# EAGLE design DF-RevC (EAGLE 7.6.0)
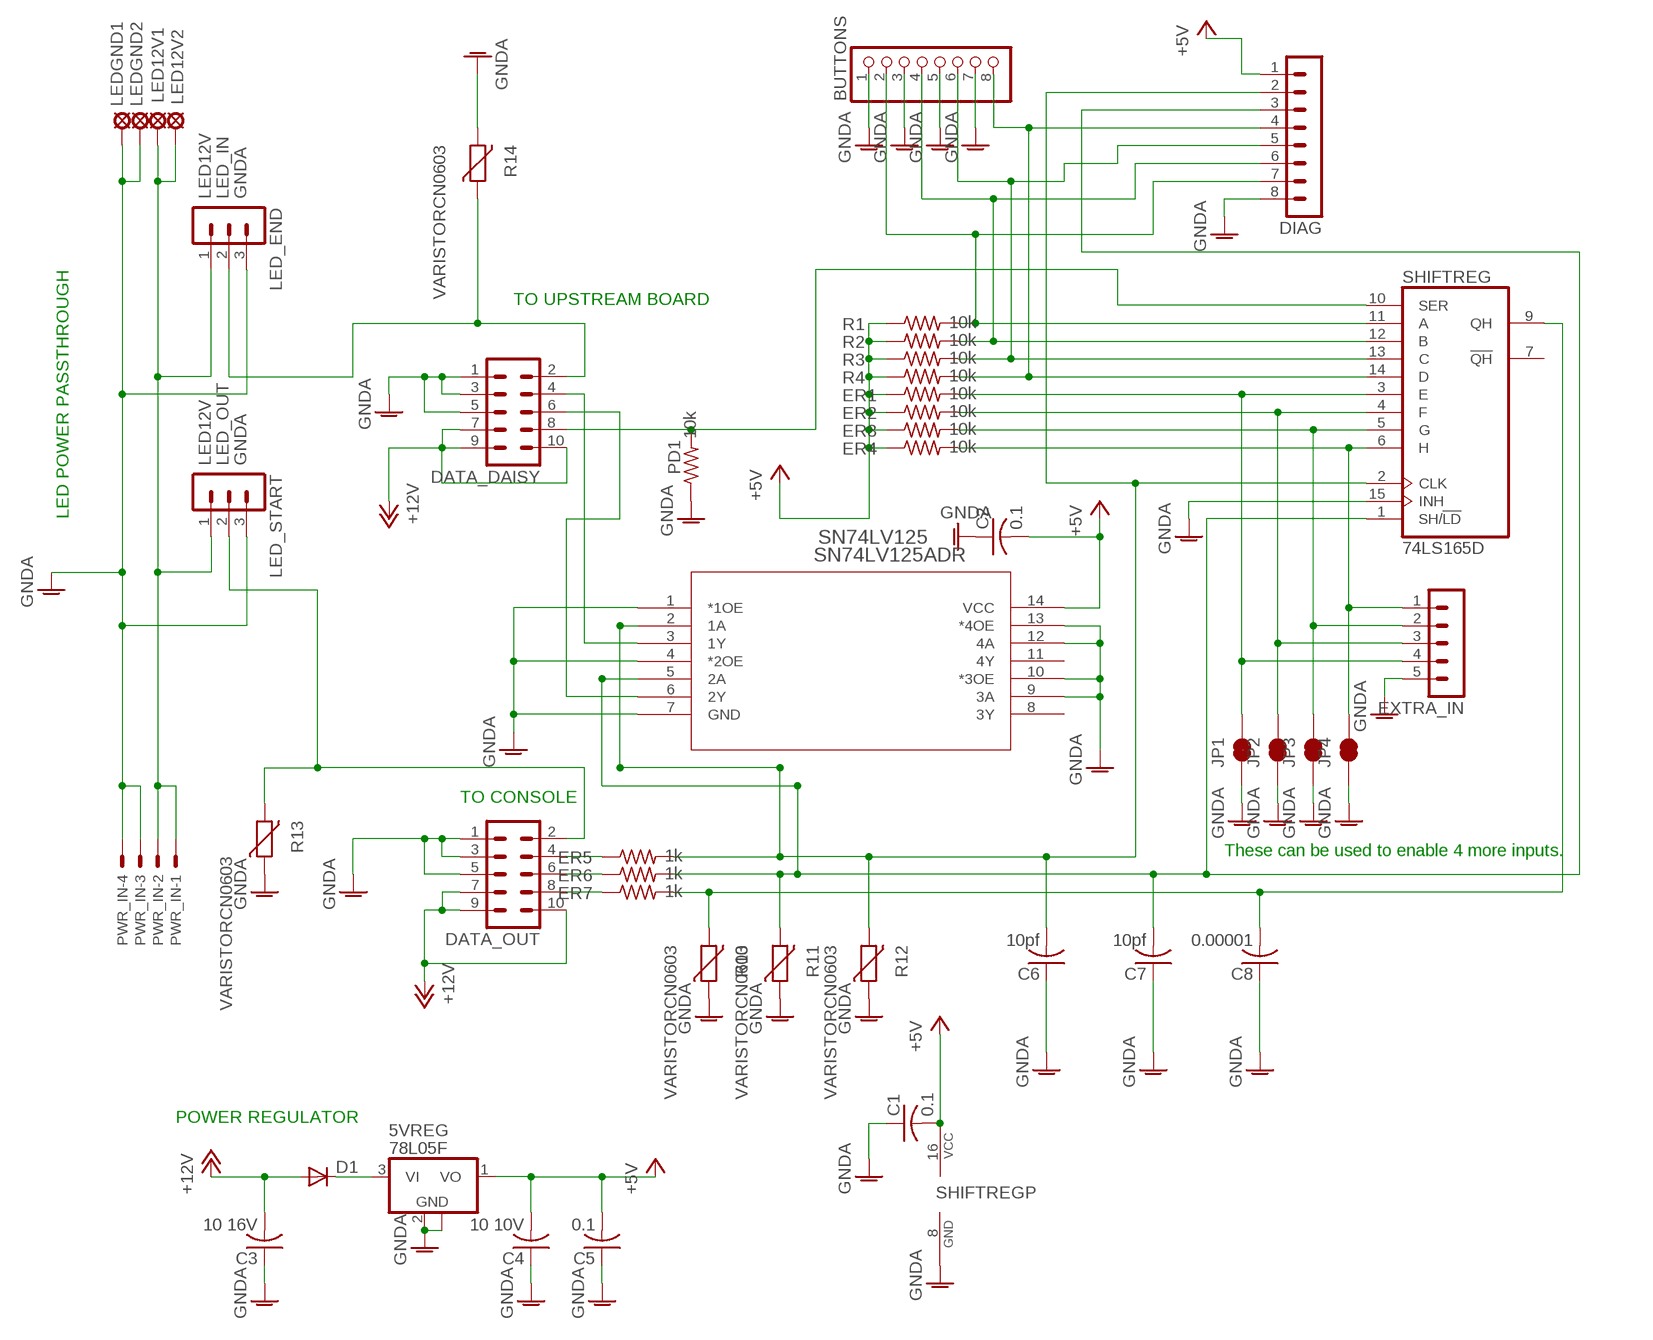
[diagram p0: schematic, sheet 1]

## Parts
5VREG  78L05F  [SOT89]
BUTTONS  SPRING-TERMINAL_8/PTSA-ZZ_2.5MM  [1X8/PTSA-ZZ_2.5MM]
C1  0.1  C-USC0603  [C0603]
C2  0.1  C-USC0603  [C0603]
C3  10 16V  C-USC0603  [C0603]
C4  10 10V  C-USC0603  [C0603]
C5  0.1  C-USC0603  [C0603]
C6  10pf  C-USC0603  [C0603]
C7  10pf  C-USC0603  [C0603]
C8  0.00001  C-USC0603  [C0603]
D1  DIODE-SOD323-R  [SOD323-R]
DATA_DAISY  MA05-2  [MA05-2]
DATA_OUT  MA05-2  [MA05-2]
DIAG  MA08-1  [MA08-1]
ER1  10k  R-US_R0603  [R0603]
ER2  10k  R-US_R0603  [R0603]
ER3  10k  R-US_R0603  [R0603]
ER4  10k  R-US_R0603  [R0603]
ER5  1k  R-US_R0603  [R0603]
ER6  1k  R-US_R0603  [R0603]
ER7  1k  R-US_R0603  [R0603]
EXTRA_IN  MA05-1  [MA05-1]
JP1  JUMPER-PAD-2-NC_BY_TRACE  [PAD-JUMPER-2-NC_BY_TRACE_YES_SILK]
JP2  JUMPER-PAD-2-NC_BY_TRACE  [PAD-JUMPER-2-NC_BY_TRACE_YES_SILK]
JP3  JUMPER-PAD-2-NC_BY_TRACE  [PAD-JUMPER-2-NC_BY_TRACE_YES_SILK]
JP4  JUMPER-PAD-2-NC_BY_TRACE  [PAD-JUMPER-2-NC_BY_TRACE_YES_SILK]
LED12V1  SE14  [SE14]
LED12V2  SE14  [SE14]
LED_END  MA03-1  [MA03-1]
LED_START  MA03-1  [MA03-1]
LEDGND1  SE14  [SE14]
LEDGND2  SE14  [SE14]
PD1  10k  R-US_R0603  [R0603]
PWR_IN  KK-156-4  [KK-156-4]
R1  10k  R-US_R0603  [R0603]
R2  10k  R-US_R0603  [R0603]
R3  10k  R-US_R0603  [R0603]
R4  10k  R-US_R0603  [R0603]
R10  VARISTORCN0603  [CT/CN0603]
R11  VARISTORCN0603  [CT/CN0603]
R12  VARISTORCN0603  [CT/CN0603]
R13  VARISTORCN0603  [CT/CN0603]
R14  VARISTORCN0603  [CT/CN0603]
SHIFTREG  74LS165D  [SO16]
SN74LV125  SN74LV125ADR  [D14]

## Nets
+5V: 5VREG.1(VO) C1.2 C2.2 C4.2 C5.2 DIAG.1 ER1.1 ER2.1 ER3.1 ER4.1 R1.1 R2.1 R3.1 R4.1 SHIFTREG.16(VCC) SN74LV125.14(VCC)
+12V: C3.2 D1.A DATA_DAISY.7 DATA_DAISY.9 DATA_DAISY.10 DATA_OUT.7 DATA_OUT.9 DATA_OUT.10
CLK: C6.2 DIAG.2 ER5.2 R12.2 SHIFTREG.2(CLK) SN74LV125.2(1A)
GNDA: 5VREG.2(GND) 5VREG.2@1(GND) BUTTONS.1 BUTTONS.3 BUTTONS.5 BUTTONS.7 C1.1 C2.1 C3.1 C4.1 C5.1 C6.1 C7.1 C8.1 DATA_DAISY.1 DATA_DAISY.3 DATA_DAISY.5 DATA_OUT.1 DATA_OUT.3 DATA_OUT.5 DIAG.8 EXTRA_IN.5 JP1.1 JP2.1 JP3.1 JP4.1 LED_END.3 LED_START.3 LEDGND1.MP LEDGND2.MP PD1.1 PWR_IN.3 PWR_IN.4 R10.1 R11.1 R12.1 R13.1 R14.2 SHIFTREG.8(GND) SHIFTREG.15(INH) SN74LV125.1(*1OE) SN74LV125.4(*2OE) SN74LV125.7(GND) SN74LV125.9(3A) SN74LV125.10(*3OE) SN74LV125.12(4A) SN74LV125.13(*4OE)
LED12V: LED12V1.MP LED12V2.MP LED_END.1 LED_START.1 PWR_IN.1 PWR_IN.2
LED_IN: DATA_DAISY.2 LED_END.2 R14.1
LED_OUT: DATA_OUT.2 LED_START.2 R13.2
LOAD: C7.2 DIAG.3 ER6.2 R11.2 SHIFTREG.1(SH/!LD) SN74LV125.5(2A)
N$1: DATA_DAISY.4 SN74LV125.3(1Y)
N$2: DATA_DAISY.8 PD1.2 SHIFTREG.10(SER)
N$4: 5VREG.3(VI) D1.C
N$6: DATA_DAISY.6 SN74LV125.6(2Y)
N$8: ER1.2 EXTRA_IN.4 JP1.2 SHIFTREG.3(E)
N$9: ER2.2 EXTRA_IN.3 JP2.2 SHIFTREG.4(F)
N$10: ER3.2 EXTRA_IN.2 JP3.2 SHIFTREG.5(G)
N$12: ER4.2 EXTRA_IN.1 JP4.2 SHIFTREG.6(H)
N$14: C8.2 ER7.2 R10.2 SHIFTREG.9(QH)
N$15: DATA_OUT.8 ER7.1
N$16: DATA_OUT.6 ER6.1
N$17: DATA_OUT.4 ER5.1
SW1: BUTTONS.2 DIAG.7 R1.2 SHIFTREG.11(A)
SW2: BUTTONS.4 DIAG.6 R2.2 SHIFTREG.12(B)
SW3: BUTTONS.6 DIAG.5 R3.2 SHIFTREG.13(C)
SW4: BUTTONS.8 DIAG.4 R4.2 SHIFTREG.14(D)
Unconnected: SHIFTREG.7(!QH) SN74LV125.8(3Y) SN74LV125.11(4Y)

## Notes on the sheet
- TO UPSTREAM BOARD
- LED POWER PASSTHROUGH
- TO CONSOLE
- These can be used to enable 4 more inputs.
- POWER REGULATOR

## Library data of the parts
5VREG = linear:78L*: POSITOIV-VOLTAGE REGULATORS Output up to 100 mA Source: Datasheet
BUTTONS = ptsa-headers:SPRING-TERMINAL_8/PTSA-ZZ_2.5MM: Spring Terminal Block Digi-Key Part Number 277-1628-ND; DIGIKEY: 277-1800-ND
C1-C8 = rcl:C-US: CAPACITOR, American symbol
D1 = diode:DIODE-: DIODE
DATA_DAISY DATA_OUT = con-lstb:MA05-2: PIN HEADER; OC_FARNELL: unknown; OC_NEWARK: unknown
DIAG = con-lstb:MA08-1: PIN HEADER; OC_FARNELL: unknown; OC_NEWARK: unknown
ER1-ER7 PD1 R1-R4 = rcl:R-US_: RESISTOR, American symbol
EXTRA_IN = con-lstb:MA05-1: PIN HEADER; OC_FARNELL: unknown; OC_NEWARK: unknown
JP1-JP4 = SparkFun-Passives:JUMPER-PAD-2-NC_BY_TRACE
LED12V1 LED12V2 LEDGND1 LEDGND2 = solpad:SE14: SOLDER PAD
LED_END LED_START = con-lstb:MA03-1: PIN HEADER; OC_FARNELL: unknown; OC_NEWARK: unknown
PWR_IN = con-molex:KK-156-4: KK 156 HEADER Source: http://www.molex.com/pdm_docs/sd/026604100_sd.pdf; OC_FARNELL: unknown; OC_NEWARK: unknown
R10-R14 = varistor:VARISTOR: VARISTOR
SHIFTREG = 74xx-us:74*165: 8-bit parallel load SHIFT REGISTER
SN74LV125 = 74125:SN74LV125ADR; 3D_LIBRARY_NAME: TI_AllParts_2012-12-25; COPYRIGHT: Copyright (C) 2015 Accelerated Designs. All rights reserved; DATASHEETURL: http://www.ti.com/lit/gpn/SN74LV125A; FAMILY_NAME: NON-INVERTING BUFFER/DRIVER; GENERIC_PART_NUMBER: SN74LV125A; INDUSTRY_STD_PKG_TYPE: SOIC; MANUFACTURER: Texas Instruments; MANUFACTURER_PART_NUMBER: SN74LV125ADR; PACKAGE_DESIGNATOR: D; PIN_COUNT: 14; VENDOR: Texas Instruments

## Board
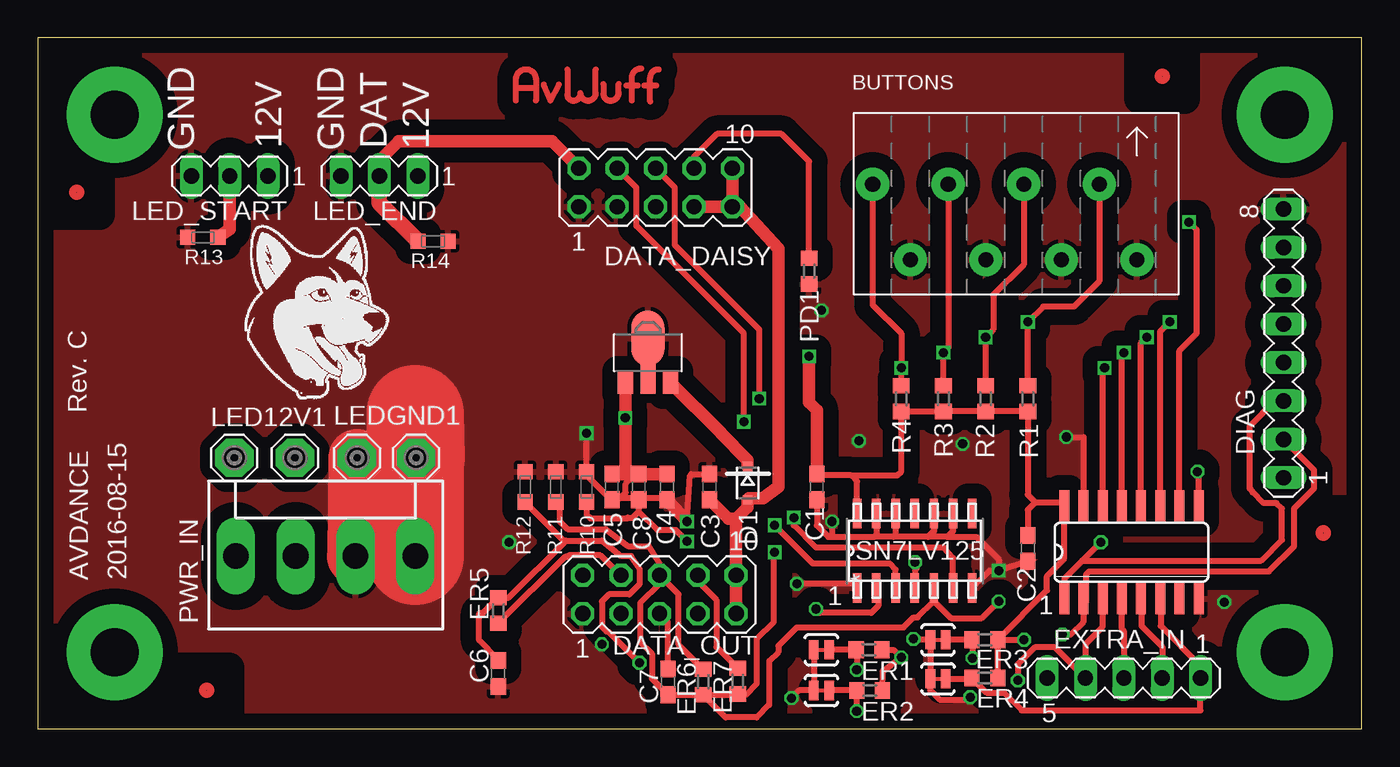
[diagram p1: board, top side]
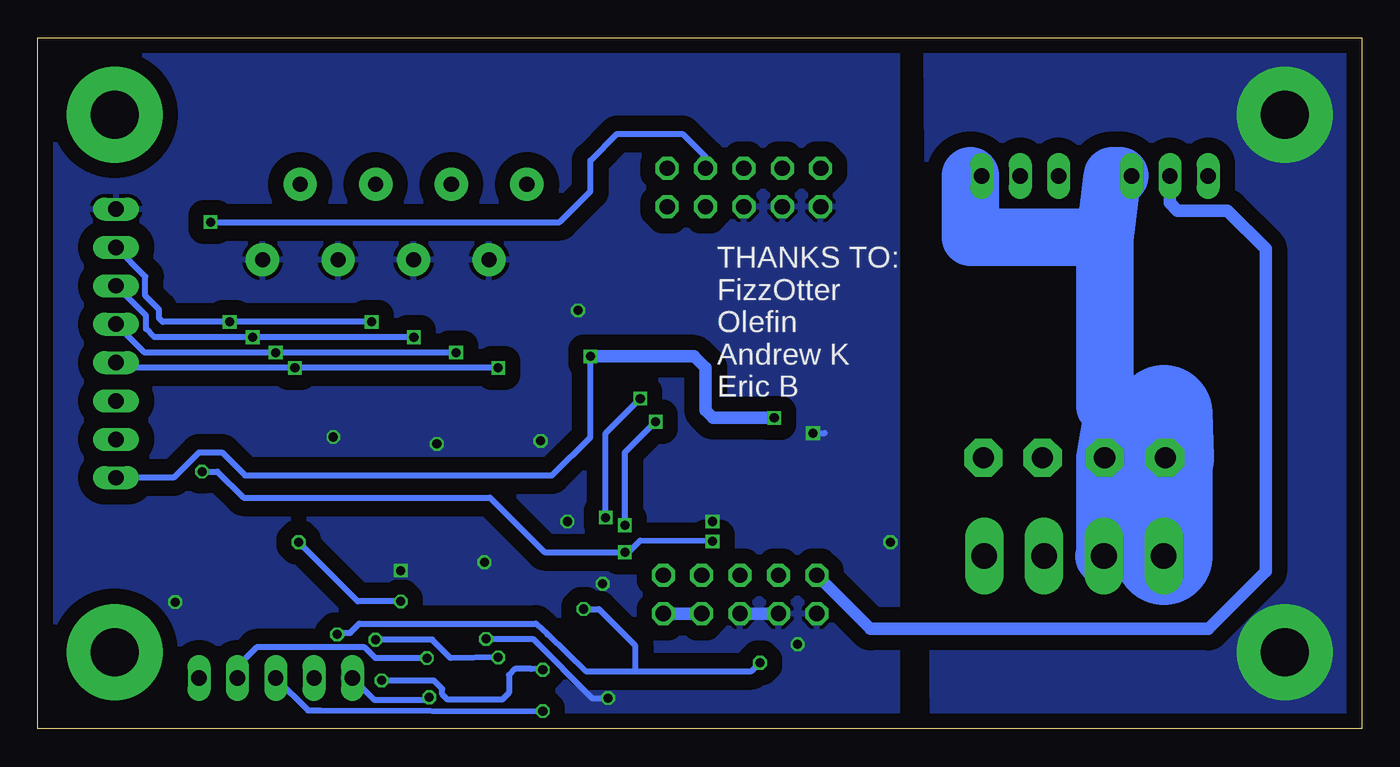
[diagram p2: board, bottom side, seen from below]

Size 87.63 x 45.72 mm. Coordinates in mm from the lower left corner, seen from the top.
Outline: 0,0 87.63,0 87.63,45.72 0,45.72 0,0
Copper layers (1*16): Top 0.035mm / dielectric 1.5mm / Bottom 0.035mm
Design rules "SeeedStudio_2layer_DRU_no_angle_20140221": minimum track width 6mil, minimum drill 12mil, track to track 6mil, track to pad 6mil, pad to pad 6mil, via to via 6mil, smd to smd 0mil, copper to edge 10mil, drill to drill 10mil, minimum pad ring 10mil, minimum via ring 6mil, stop-mask expansion 2mil, vias tented up to drill 100mil, thermal gap 10mil

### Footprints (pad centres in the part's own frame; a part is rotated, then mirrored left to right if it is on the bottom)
SOT89 = smd 1 x 1.5: 1 -1.499,-1.981; 3 1.499,-1.981 | smd 1 x 2: 2 0,-1.727 | smd 2.2 x 3.7: 2@1 0,0.94
1X8/PTSA-ZZ_2.5MM = drill 1 pad 2.2: 1 -8.75,2.5; 2 -6.25,-2.5; 3 -3.75,2.5; 4 -1.25,-2.5; 5 1.25,2.5; 6 3.75,-2.5; 7 6.25,2.5; 8 8.75,-2.5
C0603 = smd 1.1 x 1: 1 -0.85,0; 2 0.85,0
SOD323-R = smd 0.6 x 0.6: A 1.1,0; C -1.1,0
MA05-2 = drill 1.016 octagon: 1 -5.08,-1.27; 2 -5.08,1.27; 3 -2.54,-1.27; 4 -2.54,1.27; 5 0,-1.27; 6 0,1.27; 7 2.54,-1.27; 8 2.54,1.27; 9 5.08,-1.27; 10 5.08,1.27
MA08-1 = drill 1.016 long: 1 -8.89,0; 2 -6.35,0; 3 -3.81,0; 4 -1.27,0; 5 1.27,0; 6 3.81,0; 7 6.35,0; 8 8.89,0
R0603 = smd 1 x 1.1: 1 -0.85,0; 2 0.85,0
MA05-1 = drill 1.016 long: 1 -5.08,0; 2 -2.54,0; 3 0,0; 4 2.54,0; 5 5.08,0
PAD-JUMPER-2-NC_BY_TRACE_YES_SILK = smd 0.635 x 1.27: 1 -0.508,0; 2 0.508,0
SE14 = drill 1.397 pad 2.54 octagon: MP 0,0
MA03-1 = drill 1.016 long: 1 -2.54,0; 2 0,0; 3 2.54,0
KK-156-4 = drill 1.7 pad 2.184 long: 1 -5.94,0; 2 -1.98,0; 3 1.98,0; 4 5.94,0
CT/CN0603 = smd 1 x 1: 1 -1,0; 2 1,0
SO16 = smd 0.66 x 2.032: 1 -4.445,-3.073; 2 -3.175,-3.073; 3 -1.905,-3.073; 4 -0.635,-3.073; 5 0.635,-3.073; 6 1.905,-3.073; 7 3.175,-3.073; 8 4.445,-3.073; 9 4.445,3.073; 10 3.175,3.073; 11 1.905,3.073; 12 0.635,3.073; 13 -0.635,3.073; 14 -1.905,3.073; 15 -3.175,3.073; 16 -4.445,3.073
D14 = smd 1.981 x 0.559: 1 -2.464,3.81; 2 -2.464,2.54; 3 -2.464,1.27; 4 -2.464,0; 5 -2.464,-1.27; 6 -2.464,-2.54; 7 -2.464,-3.81; 8 2.464,-3.81; 9 2.464,-2.54; 10 2.464,-1.27; 11 2.464,0; 12 2.464,1.27; 13 2.464,2.54; 14 2.464,3.81

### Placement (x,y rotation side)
5VREG  40.39,24.89 0 top
BUTTONS  64.01,33.53 180 top
C1  51.56,16 90 top
C2  65.53,11.94 90 top
C3  44.45,16 270 top
C4  41.66,16 90 top
C5  38,16 90 top
C6  30.48,3.66 90 top
C7  41.71,3.1 270 top
C8  39.78,16 270 top
D1  46.99,16.26 270 top
DATA_DAISY  40.89,35.81 0 top
DATA_OUT  41.15,8.89 0 top
DIAG  82.45,25.5 90 top
ER1  55.02,5.23 180 top
ER2  55.07,2.54 180 top
ER3  62.69,5.89 180 top
ER4  62.69,3.35 180 top
ER5  30.48,7.82 90 top
ER6  44.04,3.1 270 top
ER7  46.33,3.15 270 top
EXTRA_IN  71.88,3.35 180 top
JP1  51.87,5.23 0 top
JP2  51.87,2.54 0 top
JP3  59.59,5.89 0 top
JP4  59.59,3.3 0 top
LED12V1  17.02,17.93 0 top
LED12V2  13,17.93 0 top
LED_END  22.61,36.58 180 top
LED_START  12.7,36.58 180 top
LEDGND1  25.04,17.93 0 top
LEDGND2  21.13,17.93 0 top
PD1  51.05,30.28 90 top
PWR_IN  19.05,11.43 0 top
R1  65.53,21.84 90 top
R2  62.74,21.84 90 top
R3  59.94,21.84 90 top
R4  57.15,21.84 90 top
R10  36.32,16 270 top
R11  34.29,16 270 top
R12  32.26,16 270 top
R13  10.92,32.51 0 top
R14  26.16,32.26 0 top
SHIFTREG  72.39,11.68 0 top
SN74LV125  58.05,11.78 90 top
U$1  [AVLOGO]  36.17,42.88 0 top
U$2  [FIDUCIAL]  2.59,35.51 0 top
U$3  [FIDUCIAL]  74.42,43.18 0 top
U$4  [FIDUCIAL]  85.09,12.95 0 top
U$5  [FIDUCIAL]  11.18,2.54 0 top
U$6  [AVFACE]  19,26.87 0 top

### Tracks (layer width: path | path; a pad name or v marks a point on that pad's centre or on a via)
+5V  (via drill 0.6)
  Top 0.406: 66.04,14.99 65.53,14.48 C2.2 | 66.04,14.99 67.72,14.99 SHIFTREG.16 67.94,11.25 66.8,10.11 66.8,9.16 ER3.1 | 53.85,16.76 51.65,16.76 C1.2 | 66.04,14.99 65.53,15.49 R1.1 R2.1 R3.1 R4.1 57.15,17.02 56.9,16.76 53.85,16.76 | SN74LV125.14 54.23,16.38 53.85,16.76 | ER4.1 ER3.1 | ER3.1 v65.28,5.89 | ER1.1 56.64,5.22 v57.15,4.72 55.93,3.82 ER2.1
  Top 0.813: C4.2 C5.2 38.89,17.13 v38.89,20.57 5VREG.1 | v51.05,24.64 51.05,21.59 51.56,21.08 C1.2
  Bottom 0.406: v51.05,24.64 51.05,19.3 53.59,16.76 73.91,16.76 75.44,18.29 76.96,18.29 78.64,16.61 DIAG.1 | v57.15,4.72 60.3,4.67 61.52,5.89 v65.28,5.89
  Bottom 0.813: v38.89,20.57 42.93,20.57 43.43,21.08 43.43,23.88 44.2,24.64 v51.05,24.64
+12V
  Top 0.813: 46.23,13.89 DATA_OUT.10 DATA_OUT.9 | 46.23,13.89 46.99,14.65 D1.A 47.07,15.24 48.01,15.24 49.02,16 49.02,31.75 46.48,34.54 DATA_DAISY.9 | 46.23,13.89 45.72,13.89 C3.2 | DATA_DAISY.9 DATA_DAISY.7 | DATA_DAISY.10 DATA_DAISY.9
  Bottom 0.813: DATA_OUT.9 DATA_OUT.7
CLK  (via drill 0.6)
  Top 0.406: SHIFTREG.2 69.09,8.61 | 69.09,8.61 69.09,8.13 69.39,8.43 69.39,10.21 69.6,10.41 81.48,10.41 83.16,12.09 83.16,14.58 84.48,15.9 84.48,17.12 DIAG.2 | 69.09,8.61 69.19,8.51 69.19,7.06 68.38,6.25 v67.82,6.25 | v51.51,7.92 51.77,7.67 55.17,7.67 55.63,8.13 55.63,9.2 SN74LV125.2 | R12.2 34.81,12.45 34.95,12.45 | 34.95,12.45 37.34,12.45 38.61,11.43 39.27,11.43 39.83,10.62 39.83,9.55 39.17,8.89 37.8,8.89 37.34,8.43 37.34,6.76 37.64,6.45 37.74,6.45 v39.83,4.37 39.88,4.42 39.83,4.47 | 34.95,12.45 31.18,8.67 ER5.2 29.48,7.67 29.26,7.67 29.21,7.62 29.21,5.84 30.48,4.57 C6.2
  Bottom 0.406: v67.82,6.25 67.72,6.35 66.95,6.35 66.34,6.96 54.66,6.96 53.9,6.25 51.36,3.81 48.01,3.81 | 48.01,3.81 40.39,3.81 v39.83,4.37 | v51.51,7.92 50.49,7.92 48.11,5.54 48.11,3.91 48.01,3.81
GND  (via drill 3.17 pad 6.35)
  other vias: 5.08,5.08 5.08,40.64
  pour Bottom (isolate 1.016): 0.51,45.21 28.84,44.77 28.43,0.37 0.51,0.51
GNDA  (via drill 0.6)
  Top 0.406: v42.98,13.72 43.18,16.76 43.27,16.85 C3.1 | C4.1 41.57,15.24 38.52,15.24 | v36.32,19.56 36.32,16.76 37.85,15.24 38.52,15.24 | SN74LV125.13 55.51,12.83 55.37,12.7 | SN74LV125.12 56.77,12.83 56.64,12.7 | 56.64,12.7 55.37,12.7 | SN74LV125.10 59.31,13.09 58.93,12.7 | 58.93,12.7 56.64,12.7 | 52.58,12.7 52.32,12.7 51.56,13.46 C1.1 | 52.58,12.7 55.37,12.7 | 58.17,9.31 SN74LV125.4 58.05,11.01 v58.06,11.02 58.17,10.92 58.17,10.62 | v68.07,19.3 69.22,19.3 SHIFTREG.15 | SN74LV125.9 60.58,13.08 60.2,12.7 | 60.2,12.7 58.93,12.7 | 54.23,9.31 SN74LV125.1 53.95,9.6 v50.24,9.6 | C2.1 v63.6,10.46 | 40.39,22.61 5VREG.2 5VREG.2@1 | v52.58,13.72 52.58,12.7 | C5.1 38.52,15.24 | 50.09,2.03 v49.89,2.03 50.39,2.54 JP2.1 JP1.1 | v57.96,5.94 58.01,5.89 JP3.1 JP4.1 59.08,2.54 59.69,1.93 61.47,1.93 v61.72,2.08 | SN74LV125.7 63.01,10.46 v63.6,10.46 | 60.2,12.7 62.13,12.7 63.6,11.23 v63.6,10.46 | C7.1 41.71,7.06 DATA_OUT.5 | 38.52,15.24 38.91,15.63 38.91,16.2 39.56,16.85 C8.1
  Top 0.813: C4.1 v42.98,13.72
  Top 3.81: LEDGND2.MP 21.08,11.48 PWR_IN.3
  Top 6.452: LEDGND1.MP 24.99,20.83 PWR_IN.4
  Bottom 0.406: v36.32,19.56 35.56,19.56 | v57.96,5.94 54.86,5.94 50.95,2.03 v49.89,2.03 | EXTRA_IN.5 65.38,1.93 61.98,1.93 v61.72,2.08
  Bottom 0.813: DATA_OUT.3 DATA_OUT.5
  other vias: 54.36,19.05 37.34,5.59 31.19,12.34 78.54,8.38 61.21,18.85 51.87,27.69
  pour Top (isolate 1.016): 86.87,44.7 87.12,0.51 0.88,0.24 1.08,45.04
  pour Bottom (isolate 1.016): 30.73,45.21 86.87,44.7 87.12,0.51 30.73,0.51
LED12V
  Bottom 1.016: 16,36.58 LED_START.1 | 25.91,36.58 LED_END.1
  Bottom 2.54: 17.02,21.34 16.51,20.83
  Bottom 3.81: 13.11,20.83 16.51,20.83 LED12V1.MP 17.02,11.48 PWR_IN.2 | 17.02,32.51 25.91,32.51 25.91,36.58 | 17.02,32.51 16.51,36.58 16,36.58 | 17.02,21.34 17.02,32.51
  Bottom 6.452: LED12V2.MP 13.11,20.83 PWR_IN.1
LED_IN
  Top 0.813: DATA_DAISY.2 34.04,38.86 23.88,38.86 22.61,37.59 LED_END.2
  Top 1.016: R14.1 22.61,34.81 LED_END.2
LED_OUT
  Top 0.813: R13.2 12.7,33.04 LED_START.2
  Bottom 0.813: DATA_OUT.2 32.51,6.6 10.16,6.6 6.35,10.41 6.35,31.75 8.89,34.29 12.19,34.29 12.7,34.8 LED_START.2
LOAD  (via drill 0.6)
  Top 0.406: SHIFTREG.1 67.97,8.64 67.97,9.96 69.14,11.12 | 69.14,11.12 80.97,11.12 82.35,12.5 82.35,14.58 81.99,14.94 81.13,14.94 80.42,15.65 80.42,15.7 80.21,15.9 80.21,20.02 81.89,21.69 DIAG.3 | v70.36,12.34 69.14,11.12 | 59.31,8.45 60.45,7.32 62.48,7.32 v63.6,8.43 | 59.31,8.45 58.23,7.37 57.96,7.37 57.3,6.71 50.24,6.71 49.02,5.49 49.02,5.08 48.41,4.47 48.41,1.57 47.6,0.76 45.53,0.76 ER6.2 | SN74LV125.5 59.31,8.45 | ER6.2 46.01,2.25 46.23,2.03 | ER6.2 C7.2 40.64,3.32 40.64,4.98 39.88,5.74 39.88,8.33 41.15,9.6 41.15,10.92 40.44,12.09 39.06,12.09 37.59,13.21 35.05,13.21 34.54,13.72 34.54,14.75 R11.2
  Bottom 0.406: v63.6,8.43 66.45,8.43 v70.36,12.34
N$1  (via drill 0.6)
  Top 0.406: SN74LV125.3 56.77,10.54 56.39,10.92 51.31,10.92 v48.77,13.46 | v46.74,20.32 46.74,26.16 39.62,33.27 39.62,35.81 DATA_DAISY.4
  Bottom 0.406: v48.77,13.46 48.77,18.29 v46.74,20.32
N$2  (via drill 0.6)
  Top 0.406: SHIFTREG.10 75.56,25.02 76.71,26.16 76.71,33.02 v76.2,33.53 | DATA_DAISY.8 43.43,37.85 44.96,39.37 49.23,39.37 51.05,37.54 PD1.2
  Bottom 0.406: DATA_DAISY.8 43.43,37.85 44.96,39.37 49.28,39.37 51.05,37.59 51.05,35.56 53.09,33.53 v76.2,33.53
N$4
  Top 0.813: 5VREG.3 45.21,19.58 45.21,19.56 46.99,17.78 D1.C
N$5  (via drill 3.17 pad 6.35)
  other vias: 82.55,40.64
N$6  (via drill 0.6)
  Top 0.406: SN74LV125.6 60.59,11.3 59.94,11.99 51.51,11.99 50.04,13.46 v50.04,13.97 | v47.75,21.84 47.75,26.42 42.16,32 42.16,35.81 DATA_DAISY.6
  Bottom 0.406: v50.04,13.97 50.04,19.56 v47.75,21.84
N$7  (via drill 3.17 pad 6.35)
  other vias: 82.55,5.08
N$8  (via drill 0.6)
  Top 0.406: SHIFTREG.3 70.46,8.59 70.46,6.71 69.34,5.59 EXTRA_IN.4 67.31,5.38 65.99,5.38 64.87,4.27 v64.87,3.2 | JP1.2 ER1.2 54.2,5.2 v54.2,3.91
  Bottom 0.406: v54.2,3.91 54.97,3.96 56.03,3.96 56.44,3.56 56.44,2.39 56.9,1.93 60.5,1.93 60.86,2.29 60.86,2.64 61.42,3.2 v64.87,3.2
N$9  (via drill 0.6)
  Top 0.406: SHIFTREG.4 71.73,8.59 71.73,6.66 71.88,6.5 EXTRA_IN.3 | JP2.2 ER2.2 54.22,1.49 v54.2,1.17
  Bottom 0.406: v54.2,1.17 68.94,1.22 69.75,1.22 EXTRA_IN.3
N$10  (via drill 0.6)
  Top 0.406: SHIFTREG.5 73.05,8.59 73.05,6.81 74.42,5.44 EXTRA_IN.2 | JP3.2 ER3.2 61.87,5.86 v61.87,4.67
  Bottom 0.406: v61.87,4.67 65.28,4.67 65.99,5.38 73.15,5.38 74.42,4.12 EXTRA_IN.2
N$12
  Top 0.406: SHIFTREG.6 74.32,8.59 74.32,6.81 76.96,4.17 EXTRA_IN.1 76.96,1.22 65.13,1.22 63.96,2.39 62.8,2.39 ER4.2 | ER4.2 61.79,3.3 | JP4.2 61.84,3.3 ER4.2
N$14  (via drill 0.6)
  Top 0.406: SHIFTREG.9 76.83,16.94 v76.76,17.02 | v48.77,11.68 48.72,11.63 48.72,7.06 47.6,5.94 47.6,3 46.84,2.23 46.38,2.23 46.33,2.29 ER7.2 | C8.2 39.78,14.38 | 39.78,14.38 41,13.16 42.22,13.16 v42.98,12.39 | R10.2 36.32,14.17 36.58,13.92 39.01,13.92 39.06,13.97 39.37,13.97 39.78,14.38
  Bottom 0.406: v42.98,12.39 47.75,12.45 48.51,11.68 v48.77,11.68 54.1,11.68 57.71,15.29 74.02,15.29 75.74,17.02 v76.76,17.02
N$15
  Top 0.406: DATA_OUT.8 43.69,9.75 44.91,8.53 44.91,5.42 ER7.1
N$16
  Top 0.406: ER6.1 42.42,5.57 42.42,8.89 DATA_OUT.6
N$17
  Top 0.406: DATA_OUT.4 38.56,10.16 37.24,11.48 35.15,11.48 35.05,11.38 34.89,11.38 ER5.1
SW1  (via drill 0.6)
  Top 0.406: R1.2 v65.53,26.92 66.55,27.94 68.58,27.94 70.26,29.62 BUTTONS.2 | SHIFTREG.11 74.3,26.29 v74.93,26.92
  Bottom 0.406: v65.53,26.92 v74.93,26.92 79.35,26.92 79.6,27.18 79.6,27.74 80.52,28.65 80.52,29.92 DIAG.7
SW2  (via drill 0.6)
  Top 0.406: R2.2 v62.74,25.91 63.25,26.42 63.25,28.7 65.26,30.71 BUTTONS.4 | SHIFTREG.12 73.03,25.53 v73.41,25.91
  Bottom 0.406: v62.74,25.91 v73.41,25.91 79.91,25.91 80.47,26.47 80.47,27.33 DIAG.6
SW3  (via drill 0.6)
  Top 0.406: R3.2 v59.94,24.89 60.26,25.21 BUTTONS.6 | SHIFTREG.13 71.75,24.77 v71.88,24.89
  Bottom 0.406: v59.94,24.89 v71.88,24.89 80.57,24.89 DIAG.5
SW4  (via drill 0.6)
  Top 0.406: R4.2 v57.15,23.88 57.15,26.16 55.26,28.05 BUTTONS.8 | SHIFTREG.14 70.48,23.75 v70.61,23.88
  Bottom 0.406: v57.15,23.88 v70.61,23.88 82.09,23.88 DIAG.4

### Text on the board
tNames: GND | 12V | GND | DAT | 12V | Rev. C | SN7LV125 | AVDANCE | 2016-08-15 | 1 | 1
bNames: THANKS TO: / FizzOtter / Olefin / Andrew K / Eric B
